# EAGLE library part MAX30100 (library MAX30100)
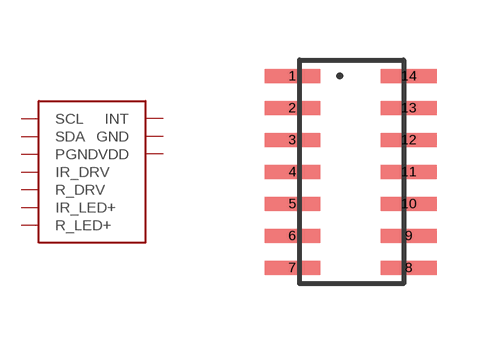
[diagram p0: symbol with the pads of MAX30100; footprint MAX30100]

Designator prefix -

## MAX30100  [MAX30100]
2  SCL
3  SDA
4  PGND
5  IR_DRV
6  R_DRV
9  R_LED+
10  IR_LED+
11  VDD
12  GND
13  INT

## Footprint MAX30100 (pad centres in mm)
smd 1.397 x 0.35: 1 -0.381,4.8; 2 -0.381,4; 3 -0.381,3.2; 4 -0.381,2.4; 5 -0.381,1.6; 6 -0.381,0.8; 7 -0.381,0; 8 2.531,0; 9 2.531,0.8; 10 2.531,1.6; 11 2.531,2.4; 12 2.531,3.2; 13 2.531,4; 14 2.531,4.8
